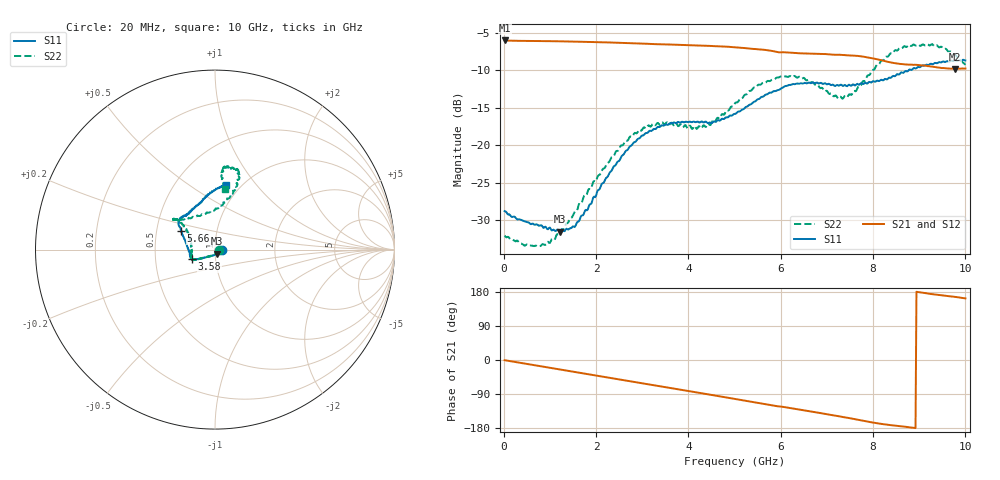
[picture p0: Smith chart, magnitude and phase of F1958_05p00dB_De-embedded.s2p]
! Integrated Device Technology
! Corporate Headquarters
! 6024 Silver Creek Valley Road
! San Jose, CA 95138  USA
! Phone:  1-408-284-8200
! Toll Free:  1-800-223-1366
! Webpage:  http://www.idt.com/
! Timing and RF Division
! 515 Groton Road, Suite 102
! Westford, MA 01886-6024
! Device:  F1958
! Description: 7-bit 0.25 dB Digital Step Attenuator
! Frequency:  0.001 -  6.000 GHz
! Package:  4x4 mm Thin QFN Plastic Package: 24 pin
! Ports:  2 RF, 12 DC
!  Pin  1  = D0
!  Pin  2  = VDD
!  Pin  3  = VMODE
!  Pin  4  = GND
!  Pin  5  = RF1  =  Port 1
!  Pin  6  = GND
!  Pin  7  = GND
!  Pin  8  = GND
!  Pin  9  = GND
!  Pin 10  = GND
!  Pin 11  = GND
!  Pin 12  = GND
!  Pin 13  = GND
!  Pin 14  = RF2  =  Port 2
!  Pin 15  = GND
!  Pin 16  = LE
!  Pin 17  = CLK
!  Pin 18  = DATA
!  Pin 19  = D6
!  Pin 20  = D5
!  Pin 21  = D4
!  Pin 22  = D3
!  Pin 23  = D2
!  Pin 24  = D1
! State:  20
! Atten State:  5.00 dB
! Voltage:  +3.30 Volts
! Current:  0.258 mA
! Data:  The device was measured on a F1958 evaluation board which has
!  individual transmission lines to the RF pins.  Data was collected
!  using a calibrated network analyzer.  The evaluation board was
!  de-embedded using Automatic Fixture Removal (AFR).
!  The reference plane is the edge of the package pin.
! Misc:
!  Action Tracker AT0419
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# GHz S dB R 50
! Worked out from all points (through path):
!   500 points, 20 MHz to 10 GHz, reference 50 ohm
!   highest |S21| = -6.05 dB at 20 MHz (marker M1); lowest = -9.8 dB at 9.78 GHz (marker M2)
!   group delay of S21, straight-line fit = 56 ps
!   lowest |S11| = -31.5 dB at 1.22 GHz (marker M3), VSWR 1.05, Z = 51.2 - j2.41 ohm
!   |S11| at or under -10 dB: start of sweep to 8.774 GHz
!   |S22| runs from -33.5 to -6.5 dB; largest |S21 - S12| = 0.0014
!   S11 on the Smith chart (normalised r, x): 20 MHz: 1.08, -0.00; 3.58 GHz: 0.77, -0.08; 5.66 GHz: 0.67, +0.15; 10 GHz: 0.85, +0.71
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0.02  -28.78 -3.2  -6.05 -0.6  -6.05 -0.5  -32.05 -4.5
0.76  -30.74 -27.4  -6.13 -15.6  -6.12 -15.6  -33.39 -45.6
1.22  -31.51 -62.2  -6.16 -25.0  -6.16 -25.0  -31.70 -90.7
1.52  -30.86 -90.9  -6.20 -31.2  -6.20 -31.2  -29.11 -114.9
1.7  -29.36 -105.1  -6.22 -34.8  -6.22 -34.8  -27.52 -125.5
2.6  -21.22 -145.8  -6.38 -53.2  -6.36 -53.3  -19.83 -150.3
2.94  -19.09 -151.3  -6.45 -60.2  -6.44 -60.3  -17.94 -152.7
3.36  -17.58 -155.3  -6.55 -68.8  -6.55 -68.9  -17.18 -156.0
3.58  -17.17 -157.7  -6.59 -73.2  -6.59 -73.4  -17.28 -160.0
4.32  -16.96 -168.2  -6.72 -88.4  -6.74 -88.5  -17.37 172.6
5.02  -15.82 169.0  -6.95 -103.1  -6.96 -103.1  -14.34 146.0
5.66  -13.31 150.9  -7.30 -116.4  -7.31 -116.4  -11.70 141.5
6.18  -11.97 144.0  -7.66 -126.4  -7.67 -126.3  -10.84 143.4
6.68  -11.67 137.6  -7.81 -136.2  -7.82 -136.1  -11.62 139.8
7.2  -12.04 130.2  -7.96 -147.1  -7.97 -147.0  -13.40 117.3
7.4  -11.99 127.5  -8.01 -151.5  -8.02 -151.4  -13.45 102.5
7.92  -11.56 115.4  -8.34 -163.3  -8.34 -163.3  -10.67 75.8
8.34  -11.02 105.1  -8.91 -171.3  -8.92 -171.4  -8.08 70.8
8.68  -10.22 96.9  -9.23 -176.0  -9.23 -175.9  -6.80 73.8
9.16  -9.27 87.6  -9.45 176.0  -9.43 176.0  -6.58 80.7
9.78  -8.69 81.2  -9.83 166.4  -9.86 166.4  -7.95 83.9
10  -8.71 80.5  -9.78 162.5  -9.81 162.6  -9.30 80.4
